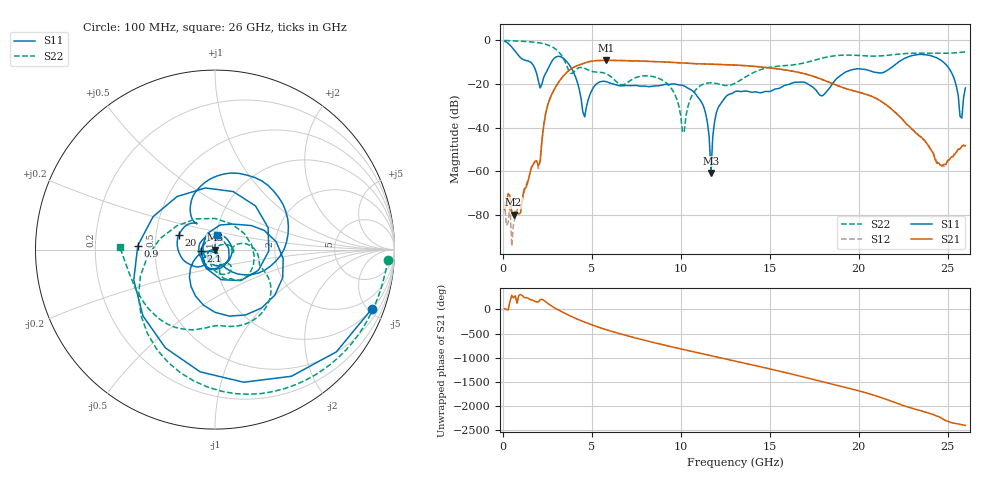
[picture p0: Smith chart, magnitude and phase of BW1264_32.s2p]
!Keysight Technologies,N5245B,MY57181159,A.13.60.06
!Date: Friday, December 18, 2020 23:53:36
!Correction: S11(Full 2 Port(1,2))
!S21(Full 2 Port(1,2))
!S12(Full 2 Port(1,2))
!S22(Full 2 Port(1,2))
!S2P File: Measurements: S11, S21, S12, S22:
# Hz S  dB  R 50
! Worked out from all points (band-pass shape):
!   260 points, 100 MHz to 26 GHz, reference 50 ohm
!   highest |S21| = -9.40 dB at 5.8 GHz (marker M1); lowest = -79.7 dB at 600 MHz (marker M2)
!   |S21| within 3 dB of the highest: 4.018 GHz to 14.53 GHz (10.52 GHz wide, 113 % of centre)
!   lowest |S11| = -60.7 dB at 11.7 GHz (marker M3), VSWR 1.00, Z = 50 - j0.0908 ohm
!   |S11| at or under -10 dB: 1.52 GHz to 2.745 GHz (1.225 GHz wide, 57.5 % of centre); 3.6 GHz to 22.26 GHz (18.66 GHz wide, 144 % of centre); 24.73 GHz to end of sweep
!   |S22| runs from -42.3 to -0.3 dB; largest |S21 - S12| = 0.00044
!   S11 on the Smith chart (normalised r, x): 100 MHz: 1.01, -5.24; 900 MHz: 0.40, +0.02; 2.1 GHz: 0.85, -0.01; 20 GHz: 0.66, +0.11; 26 GHz: 1.01, +0.16
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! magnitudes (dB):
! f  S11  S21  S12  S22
! 100 MHz  -0.6  -77.4  -73.8  -0.3
! 600 MHz  -4.2  -79.7  -83.8  -0.5
! 900 MHz  -7.3  -79.5  -75.9  -0.6
! 2.1 GHz  -22.0  -55.5  -54.5  -1.5
! 2.5 GHz  -13.9  -30.4  -30.4  -2.3
! 3.3 GHz  -7.9  -17.5  -17.5  -7.1
! 4.5 GHz  -33.0  -10.9  -10.9  -12.7
! 5.8 GHz  -19.1  -9.4  -9.4  -15.4
! 8.8 GHz  -20.9  -10.0  -10.0  -17.7
! 10.1 GHz  -20.8  -10.6  -10.6  -42.3
! 11.2 GHz  -28.9  -11.0  -11.0  -20.5
! 11.5 GHz  -37.7  -11.1  -11.1  -19.7
! 11.7 GHz  -60.7  -11.1  -11.1  -19.6
! 12 GHz  -33.3  -11.2  -11.2  -19.9
! 13.1 GHz  -23.5  -11.5  -11.5  -19.6
! 17.4 GHz  -21.5  -16.5  -16.5  -9.6
! 20 GHz  -13.2  -23.9  -23.9  -7.2
! 21.7 GHz  -13.5  -30.6  -30.6  -7.0
! 24.5 GHz  -8.7  -56.1  -57.3  -6.1
! 25.4 GHz  -18.5  -52.2  -51.5  -6.0
! 25.7 GHz  -34.9  -49.8  -49.6  -5.8
! 26 GHz  -21.9  -48.3  -48.5  -5.5
